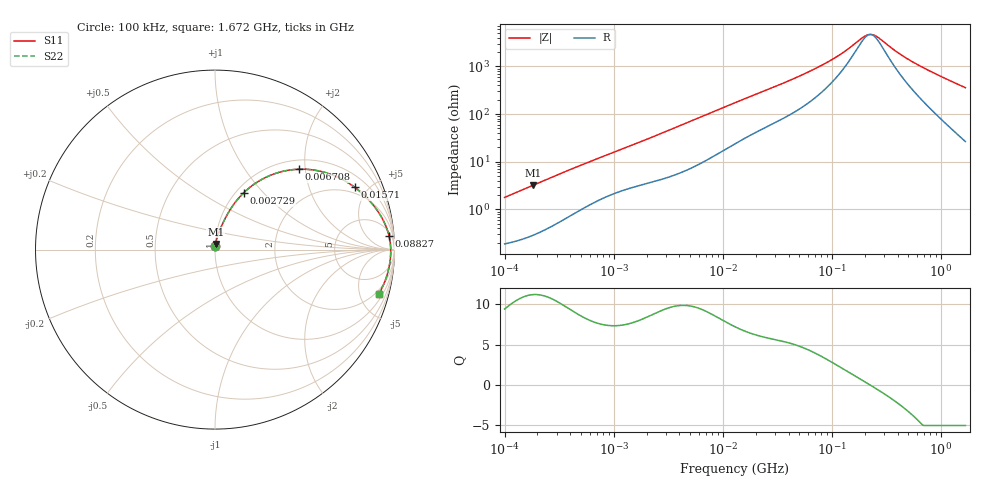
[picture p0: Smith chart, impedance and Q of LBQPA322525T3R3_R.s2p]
! LBQPA322525T3R3_R  S-PARAMETER MODEL  ( General Type )
! Model Generated by TAIYO YUDEN Corporation (http://www.ty-top.com)
! Version 1.0
! TAIYO YUDEN Control No. 191025NI43SB-FBB
! Copyright(c) 2019 TAIYO YUDEN CO.,LTD. All Rights Reserved.
! Product Description (link to TY-COMPAS)
! https://ds.yuden.co.jp/TYCOMPAS/or/detail?pn=LBQPA322525T3R3MR&u=M
! Products Name : Inductors
! Characteristics :
!  Inductance : 3.3 uH , SRF(min) : 160 MHz , DC Resistance(max) : 0.1235 Ohm
!  Rated Current : Saturation :2000 mA , Temp Rise : 850 mA (20 degC)
!  Case Size : 3.2 x 2.5 / 0.126 x 0.098 [mm/inch] , Thickness : 2.5 / 0.098 [mm/inch]
!  (Conditions: Temperature = 25 degC , DC Bias Current/Voltage = 0A / 0V)
! External Node Assignments :
!  1  o---GGG---o  2
! GND o---------o GND
! Frequency Range : 0.1MHz  -  1672.468556MHz  [ 402 STEP ]
# MHz S RI R 50
! Freq[MHz].  S11 Real  S11 Imag  S21 Real  S21 Imag  S12 Real  S12 Imag  S22 Real  S22 Imag
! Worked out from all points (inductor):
!   401 points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, 100 kHz to 1.672 GHz, reference 50 ohm
!   read as one part in series: L = 2.82 uH near 105 kHz
!   highest Q = 11.2 at 183.6 kHz (marker M1), where L = 2.8 uH
!   self-resonance near 224.4 MHz
!   S11 on the Smith chart (normalised r, x): 100 kHz: 1.00, +0.04; 2.729 MHz: 1.09, +0.78; 6.708 MHz: 1.20, +1.86; 15.71 MHz: 1.61, +4.11; 88.27 MHz: 8, +23; 1.672 GHz: 1.53, -7.14
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0.1  0.0022 0.0177  0.9978 -0.0177  0.9978 -0.0177  0.0022 0.0177
0.183637  0.00392 0.0321  0.9961 -0.0321  0.9961 -0.0321  0.00392 0.0321
0.509815  0.017 0.0833  0.983 -0.0833  0.983 -0.0833  0.017 0.0833
1.348181  0.0632 0.186  0.9368 -0.186  0.9368 -0.186  0.0632 0.186
2.599112  0.1493 0.3055  0.8507 -0.3055  0.8507 -0.3055  0.1493 0.3055
2.728612  0.1594 0.3157  0.8406 -0.3157  0.8406 -0.3157  0.1594 0.3157
4.125099  0.2748 0.3985  0.7252 -0.3985  0.7252 -0.3985  0.2748 0.3985
6.708143  0.4694 0.4479  0.5306 -0.4479  0.5306 -0.4479  0.4694 0.4479
12.9324  0.7241 0.383  0.2759 -0.383  0.2759 -0.383  0.7241 0.383
15.70891  0.7794 0.3467  0.2206 -0.3467  0.2206 -0.3467  0.7794 0.3467
29.55728  0.8976 0.2273  0.1024 -0.2273  0.1024 -0.2273  0.8976 0.2273
65.93127  0.9604 0.1085  0.0396 -0.1085  0.0396 -0.1085  0.9604 0.1085
88.26574  0.9696 0.0765  0.0304 -0.0765  0.0304 -0.0765  0.9696 0.0765
127.1066  0.9758 0.0433  0.0242 -0.0433  0.0242 -0.0433  0.9758 0.0433
192.159  0.9787 0.0113  0.0213 -0.0113  0.0213 -0.0113  0.9787 0.0113
216.9965  0.9791 0.00244  0.0209 -0.00244  0.0209 -0.00244  0.9791 0.00244
233.4146  0.9792 -0.00288  0.0208 0.00288  0.0208 0.00288  0.9792 -0.00288
257.2537  0.9792 -0.01  0.0208 0.01  0.0208 0.01  0.9792 -0.01
336.1274  0.9786 -0.0303  0.0214 0.0303  0.0214 0.0303  0.9786 -0.0303
449.9918  0.9765 -0.0548  0.0235 0.0548  0.0235 0.0548  0.9765 -0.0548
632.4441  0.9715 -0.0892  0.0285 0.0892  0.0285 0.0892  0.9715 -0.0892
1672.469  0.9118 -0.2489  0.0882 0.2489  0.0882 0.2489  0.9118 -0.2489
